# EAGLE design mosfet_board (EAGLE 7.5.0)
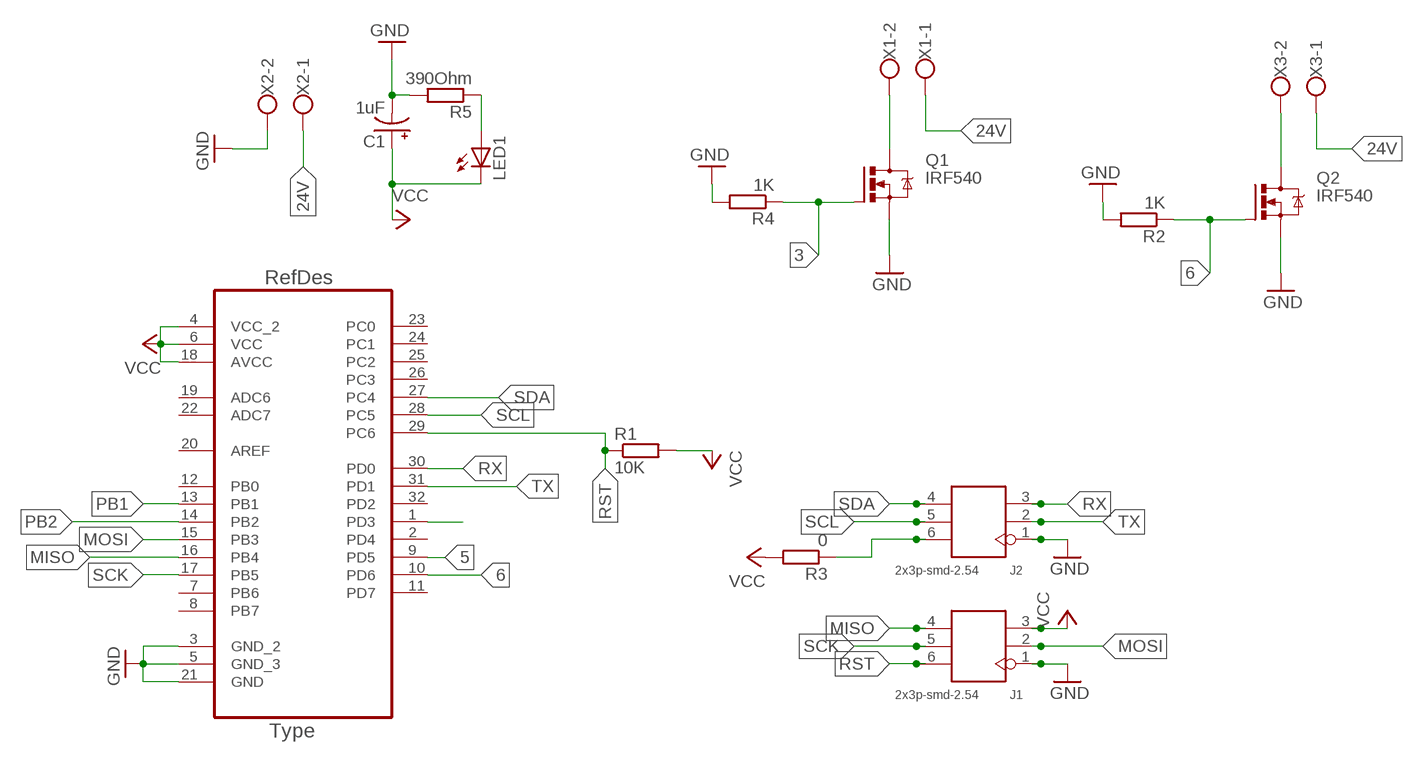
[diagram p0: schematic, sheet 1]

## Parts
C1  1uF  CAP_POL1206-KIT  [EIA3216-KIT]
J1  2x3p-smd-2.54  SMD-BLUE-FEMALE-HEADER-VERT(2X3P-2.54)  [H2X3-SMD-2.54]
J2  2x3p-smd-2.54  SMD-BLUE-FEMALE-HEADER-VERT(2X3P-2.54)  [H2X3-SMD-2.54]
LED1  LEDP-LCC-2  [P-LCC-2]
Q1  IRF540  [TO220BV]
Q2  IRF540  [TO220BV]
R1  10K  R-EU_M1206  [M1206]
R2  1K  R-EU_M1206  [M1206]
R3  0  R-EU_M1206  [M1206]
R4  1K  R-EU_M1206  [M1206]
R5  390Ohm  R-EU_M1206  [M1206]
U1  ATMEGA328P-AU  [QFP80P900X900X120-32N]
X1  W237-102  [W237-102]
X2  W237-102  [W237-102]
X3  W237-102  [W237-102]

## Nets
3: Q1.G R4.1 U1.1(PD3)
5: U1.9(PD5)
6: Q2.G R2.1 U1.10(PD6)
24V: X1.1 X2.1 X3.1
GND: C1.C(-) J1.1 J2.1 Q1.S Q2.S R2.2 R4.2 R5.2 U1.3(GND_2) U1.5(GND_3) U1.21(GND) X2.2
MISO: J1.4 U1.16(PB4)
MOSI: J1.2 U1.15(PB3)
N$1: Q1.D X1.2
N$2: Q2.D X3.2
N$3: J2.6 R3.1
N$5: LED1.A R5.1
PB1: U1.13(PB1)
PB2: U1.14(PB2)
RST: J1.6 R1.1 U1.29(PC6)
RX: J2.3 U1.30(PD0)
SCK: J1.5 U1.17(PB5)
SCL: J2.5 U1.28(PC5)
SDA: J2.4 U1.27(PC4)
TX: J2.2 U1.31(PD1)
VCC: C1.A(+) J1.3 LED1.C R1.2 R3.2 U1.4(VCC_2) U1.6(VCC) U1.18(AVCC)
Unconnected: U1.2(PD4) U1.7(PB6) U1.8(PB7) U1.11(PD7) U1.12(PB0) U1.19(ADC6) U1.20(AREF) U1.22(ADC7) U1.23(PC0) U1.24(PC1) U1.25(PC2) U1.26(PC3) U1.32(PD2)

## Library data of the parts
C1 = SparkFun-Passives:CAP_POL: Capacitor Polarized
J1 J2 = Seeed-OPL-Connector:SMD-BLUE-FEMALE-HEADER-VERT(2X3P-2.54): 320030035; MPN: F185-1203A1BMYA1
LED1 = led:LED: LED
Q1 Q2 = transistor-power:IRF540: HEXFET Power MOSFET
R1-R5 = rcl:R-EU_: RESISTOR, European symbol
U1 = ATMEGA328P-AU:ATMEGA328P-AU; DESCRIPTION: 8-bit Microcontroller with In-System Programmable Flash; MPN: ATMEGA328P-AU; OC_FARNELL: 1715486; OC_NEWARK: 14R4631; PACKAGE: TQFP-32; SUPPLIER: Atmel
X1-X3 = con-wago-500:W237-102: WAGO SCREW CLAMP; MPN: 237-102; OC_FARNELL: unknown; OC_NEWARK: 70K9898

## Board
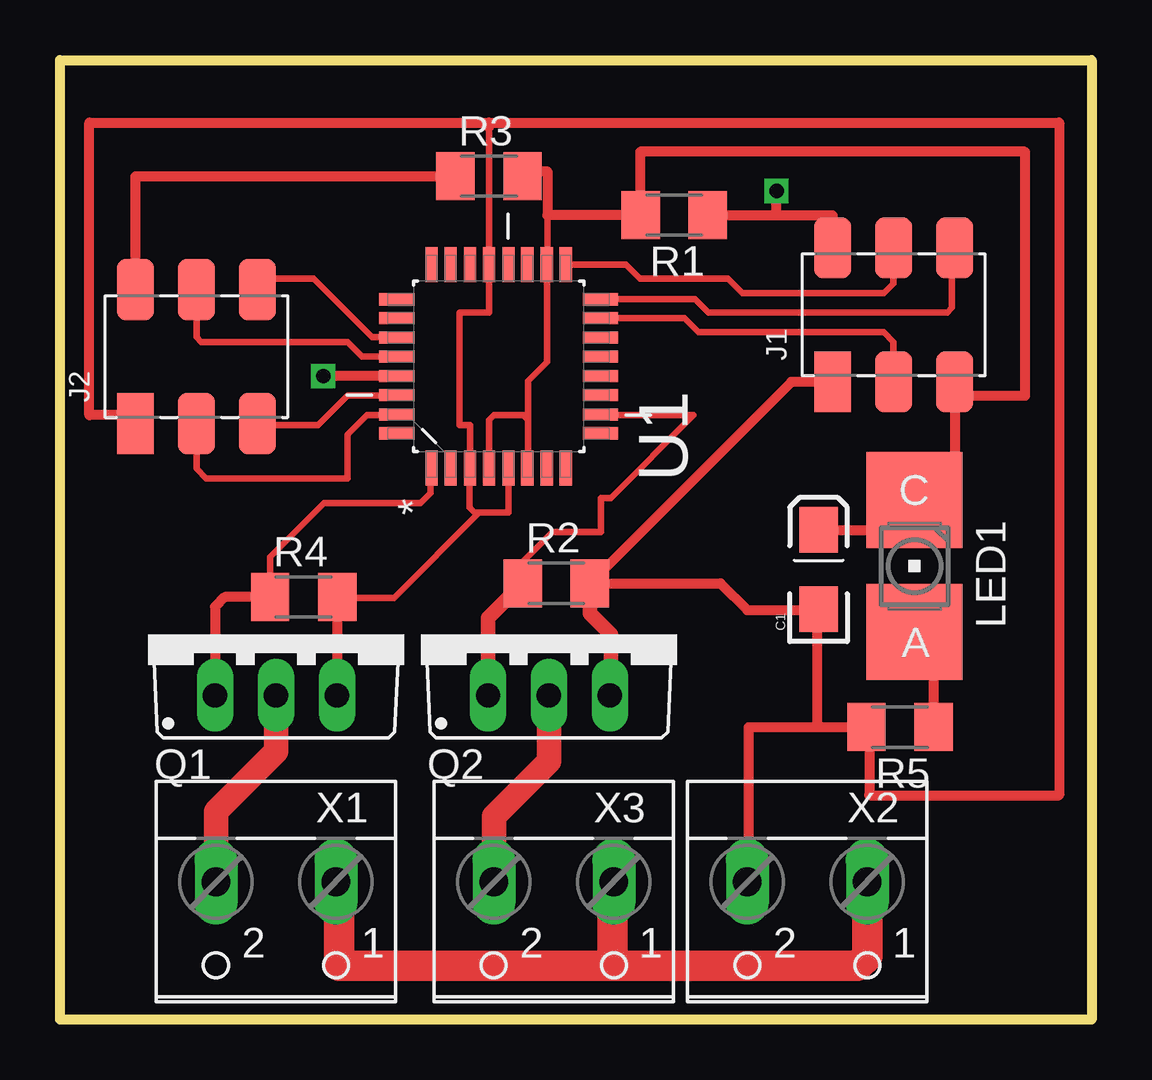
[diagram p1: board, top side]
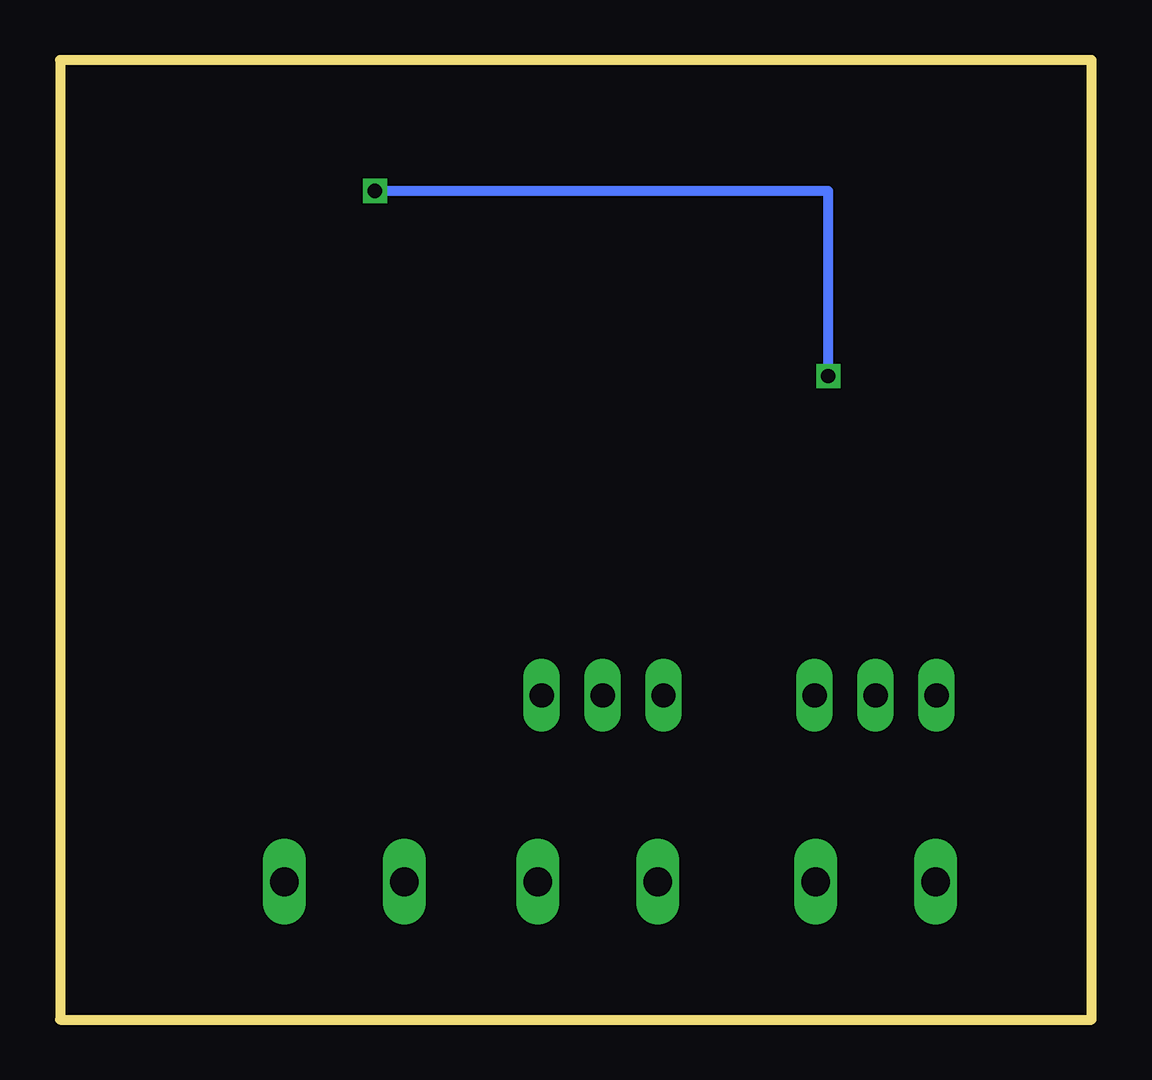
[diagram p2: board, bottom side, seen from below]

Size 43 x 40 mm. Coordinates in mm from the lower left corner, seen from the top.
Outline: 0,0 43,0 43,40 0,40 0,0
Copper layers (1*16): Top 0.035mm / dielectric 1.5mm / Bottom 0.035mm
Design rules "default *": minimum track width 10mil, minimum drill 24mil, track to track 12mil, track to pad 12mil, pad to pad 13mil, via to via 13mil, smd to smd 13mil, copper to edge 40mil, drill to drill 8mil, minimum pad ring 10mil, minimum via ring 8mil, stop-mask expansion 4mil, vias tented up to drill 0mil, thermal gap 10mil
Milling: 4 lines

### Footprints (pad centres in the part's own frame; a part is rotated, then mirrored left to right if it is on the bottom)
EIA3216-KIT = smd 1.9 x 1.6: A 1.65,0; C -1.65,0
H2X3-SMD-2.54 = smd 2.54 x 1.524: 1 -2.794,2.54; 2 -2.794,0; 3 -2.794,-2.54; 4 2.794,-2.54; 5 2.794,0; 6 2.794,2.54
P-LCC-2 = smd 4 x 4: A 0,2.75; C 0,-2.75
TO220BV = drill 1.016 long: D 0,-2.54; G -2.54,-2.54; S 2.54,-2.54
M1206 = smd 1.6 x 2: 1 -1.4,0; 2 1.4,0
QFP80P900X900X120-32N = smd 1.473 x 0.508: 1 -4.242,2.794; 2 -4.242,2.007; 3 -4.242,1.194; 4 -4.242,0.406; 5 -4.242,-0.406; 6 -4.242,-1.194; 7 -4.242,-2.007; 8 -4.242,-2.794; 17 4.242,-2.794; 18 4.242,-2.007; 19 4.242,-1.194; 20 4.242,-0.406; 21 4.242,0.406; 22 4.242,1.194; 23 4.242,2.007; 24 4.242,2.794 | smd 0.508 x 1.473: 9 -2.794,-4.242; 10 -2.007,-4.242; 11 -1.194,-4.242; 12 -0.406,-4.242; 13 0.406,-4.242; 14 1.194,-4.242; 15 2.007,-4.242; 16 2.794,-4.242; 25 2.794,4.242; 26 2.007,4.242; 27 1.194,4.242; 28 0.406,4.242; 29 -0.406,4.242; 30 -1.194,4.242; 31 -2.007,4.242; 32 -2.794,4.242
W237-102 = drill 1.194 long: 1 -2.5,-1.27; 2 2.5,-1.27

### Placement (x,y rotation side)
C1  31.62,18.76 90 top
J1  34.75,29.38 90 top
J2  5.69,27.64 90 top
LED1  35.62,18.9 180 top
Q1  9,16.05 0 top
Q2  20.38,16.05 0 top
R1  25.6,33.53 180 top
R2  20.69,18.19 0 top
R3  17.88,35.15 0 top
R4  10.16,17.61 0 top
R5  35.01,12.19 180 top
U1  18.29,27.23 90 top
X1  9,4.47 180 top
X2  31.15,4.47 180 top
X3  20.59,4.47 180 top

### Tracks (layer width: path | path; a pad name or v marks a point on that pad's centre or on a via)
3
  Top 0.279: R4.1 8.76,19.28 11.02,21.54 15.04,21.54 15.44,21.95 15.44,22.94 U1.1
  Top 0.406: R4.1 6.87,17.61 6.46,17.21 Q1.G
6
  Top 0.279: R2.1 19.3,18.2 19.3,19.1 20.52,20.32 22.55,20.32 22.55,21.74 22.96,21.74 26.42,25.2 22.55,25.2 U1.10
  Top 0.61: Q2.G 17.84,16.74 R2.1
24V
  Top 1.27: 23.02,5.74 X3.1 23.02,5.68 23.02,2.23 | X1.1 11.64,5.6 11.64,2.23 23.02,2.23 | 23.02,2.23 33.25,2.23 33.65,2.64 X2.1
GND
  Top 0.279: 11.38,17.8 R4.2 | 17.88,37.19 U1.21 17.88,29.46 16.66,29.46 16.66,24.79 17.09,24.79 U1.3 17.07,22.96 17.07,21.34 17.27,21.13 17.48,21.13 | U1.5 18.69,21.13 17.48,21.13 | 11.65,17.58 13.92,17.58 17.48,21.13
  Top 0.406: 11.65,17.58 arc-45 R4.2 11.56,13.55 arc-45 Q1.S | X2.2 28.71,5.8 28.71,12.19 31.56,12.19 | 31.56,12.19 R5.2 33.73,12.19 33.73,9.35 41.66,9.35 41.66,37.39 17.88,37.39 | C1.C 31.56,17.05 31.56,12.19 | 17.88,37.19 17.88,37.39 | J1.1 30.48,26.58 R2.2 27.53,18.19 28.65,17.07 31.58,17.07 | J2.1 3.15,25.2 1.22,25.2 1.22,37.39 17.88,37.39
  Top 0.61: 31.58,17.07 C1.C | R2.2 22.09,16.93 22.96,16.05 22.96,13.55 Q2.S
MISO
  Top 0.279: U1.16 26.47,30.02 27.03,29.46 36.98,29.46 37.19,29.67 37.19,32.07 J1.4
MOSI
  Top 0.279: U1.15 26.04,29.23 26.62,28.65 34.34,28.65 34.75,28.25 J1.2
N$1
  Top 1.016: X1.2 6.5,8.68 9,11.18 Q1.D
N$2
  Top 1.016: X3.2 18.09,8.47 20.38,10.77 Q2.D
N$3
  Top 0.406: J2.6 3.15,35.15 R3.1
N$5
  Top 0.406: LED1.A 36.01,16.15 36.41,15.74 R5.1
RST  (via drill 0.6)
  Top 0.406: U1.29 v10.97,26.82 | J1.6 32.21,33.53 R1.1 29.87,33.53 v29.87,34.54
  Bottom 0.406: v10.97,26.82 10.97,34.54 v29.87,34.54
RX
  Top 0.279: U1.30 14.02,26.01 11.99,26.01 10.77,24.79 8.28,24.79 J2.3
SCK
  Top 0.279: U1.17 23.6,31.47 24.18,30.89 27.84,30.89 28.45,30.28 34.34,30.28 34.75,30.68 J1.5
SCL
  Top 0.279: U1.28 12.6,27.64 11.99,28.25 5.89,28.25 5.69,28.45 J2.5
SDA
  Top 0.279: U1.27 14.02,28.45 13.01,28.45 10.57,30.89 8.69,30.89 J2.4
TX
  Top 0.279: U1.31 14.02,25.2 12.8,25.2 11.99,24.38 11.99,22.55 6.1,22.55 5.69,22.96 J2.2
VCC
  Top 0.279: U1.18 20.3,27.41 19.51,26.62 19.51,24.99 | 19.51,24.99 19.51,23.01 U1.6 | U1.4 17.88,24.99 18.09,25.2 19.3,25.2 19.51,24.99 | 20.32,31.47 20.32,33.53
  Top 0.406: 37.45,26.42 37.31,26.56 37.31,22.13 36.49,22.13 | J1.3 37.29,26.01 40.23,26.01 40.23,36.17 24.18,36.17 24.18,33.53 R1.2 20.32,33.53 20.32,35.36 19.28,35.36 R3.2 | 20.32,31.47 U1.18 | C1.A 34.38,20.41 LED1.C
  Top 0.61: LED1.C 36.49,22.13 36.72,22.26 | 37.31,26.56 J1.3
